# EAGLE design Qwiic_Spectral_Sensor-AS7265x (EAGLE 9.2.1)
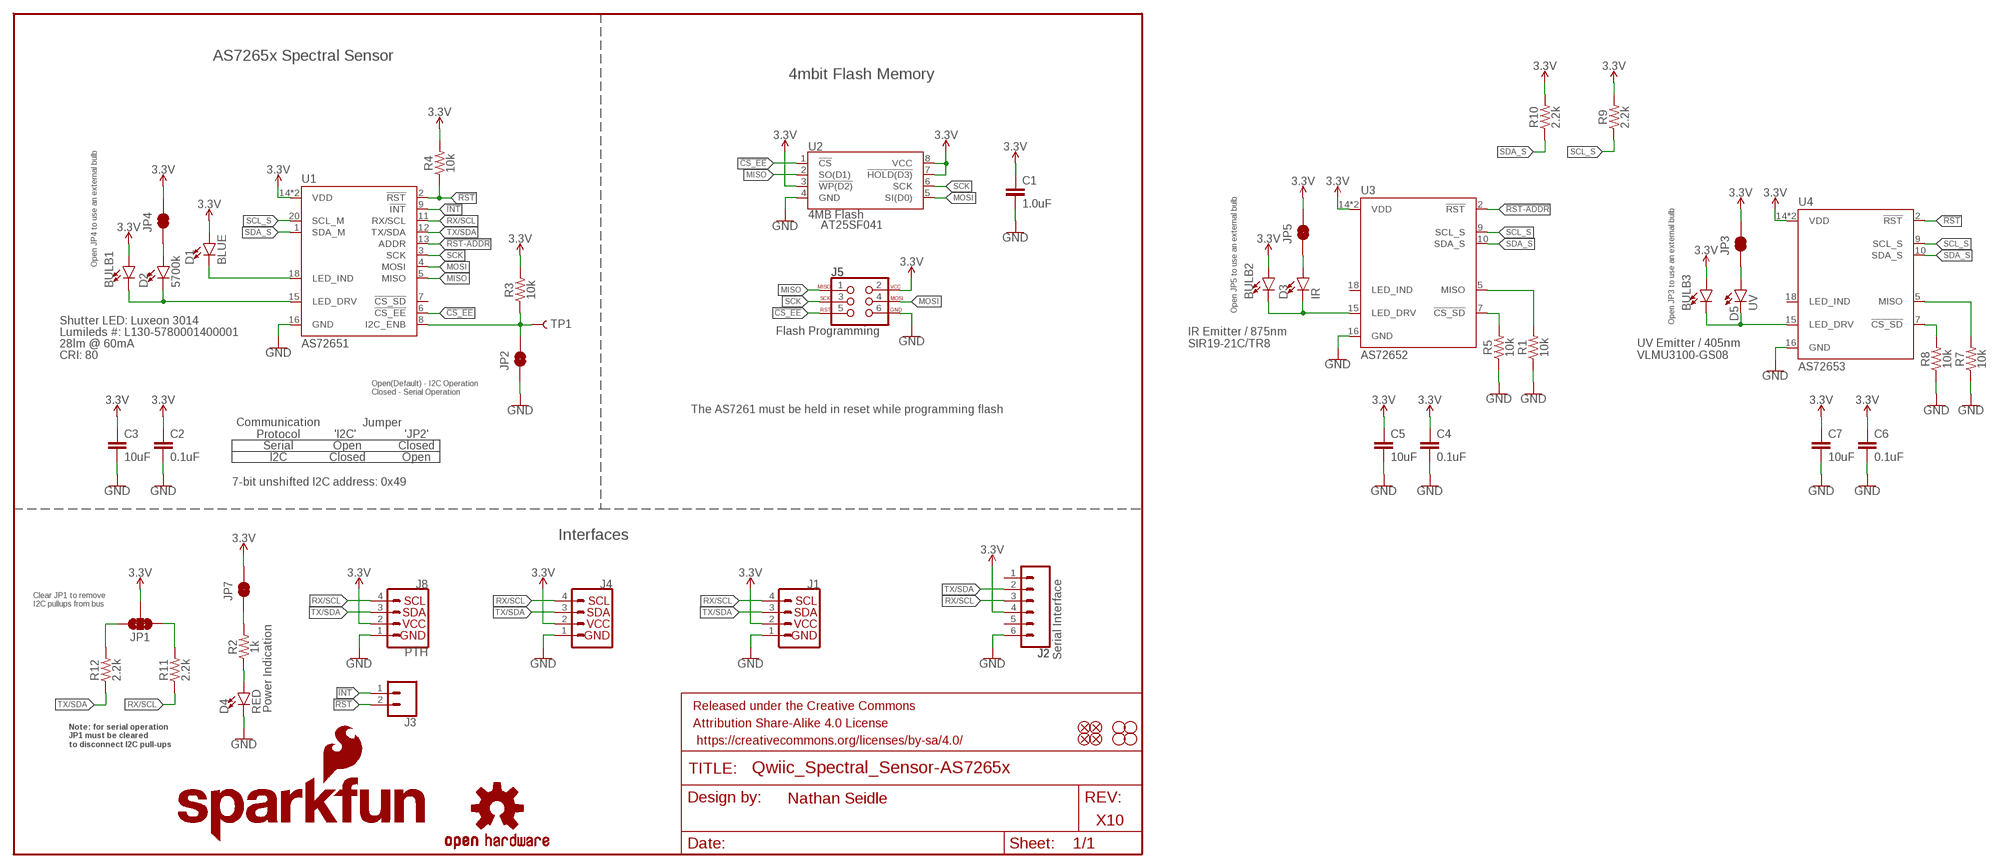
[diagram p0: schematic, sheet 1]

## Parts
BULB1  LEDNS  [LED_5MM_NOSILK]
BULB2  LEDNS  [LED_5MM_NOSILK]
BULB3  LEDNS  [LED_5MM_NOSILK]
C1  1.0uF  1.0UF-0603-16V-10%  [0603]
C2  0.1uF  0.1UF-0603-25V-(+80/-20%)  [0603]
C3  10uF  10UF-0603-6.3V-20%  [0603]
C4  0.1uF  0.1UF-0603-25V-(+80/-20%)  [0603]
C5  10uF  10UF-0603-6.3V-20%  [0603]
C6  0.1uF  0.1UF-0603-25V-(+80/-20%)  [0603]
C7  10uF  10UF-0603-6.3V-20%  [0603]
D1  BLUE  LED-BLUE0603  [LED-0603]
D2  5700k  LED-WHITE3014  [SUPER_BRIGHT_SMD_LED_3014]
D3  IR  LED-IR0603  [LED-0603]
D4  RED  LED-RED0603  [LED-0603]
D5  UV  LED-UVPLCC  [PLCC-2]
FD1  FIDUCIAL1X2  [FIDUCIAL-1X2]
FD2  FIDUCIAL1X2  [FIDUCIAL-1X2]
FD3  FIDUCIAL1X2  [FIDUCIAL-1X2]
FD4  FIDUCIAL1X2  [FIDUCIAL-1X2]
FRAME1  FRAME-LETTER  [CREATIVE_COMMONS]
H1  STAND-OFF  [STAND-OFF]
H2  STAND-OFF  [STAND-OFF]
H3  STAND-OFF  [STAND-OFF]
H4  STAND-OFF  [STAND-OFF]
J1  QWIIC_CONNECTORJS-1MM  [1X04_1MM_RA]
J2  Serial Interface  CONN_06NO_SILK_FEMALE_PTH  [1X06_NO_SILK]
J3  CONN_021X02_NO_SILK  [1X02_NO_SILK]
J4  QWIIC_CONNECTORJS-1MM  [1X04_1MM_RA]
J5  Flash Programming  AVR_SPI_PROG_3X2TESTPOINTS  [2X3_TEST_POINTS]
J8  PTH  I2C_STANDARD_NO_SILK  [1X04_NO_SILK]
JP1  JUMPER-SMT_3_2-NC_TRACE_SILK  [SMT-JUMPER_3_2-NC_TRACE_SILK]
JP2  JUMPER-SMT_2_NO_SILK  [SMT-JUMPER_2_NO_SILK]
JP3  JUMPER-SMT_2_NC_TRACE_NO-SILK  [SMT-JUMPER_2_NC_TRACE_NO-SILK]
JP4  JUMPER-SMT_2_NC_TRACE_NO-SILK  [SMT-JUMPER_2_NC_TRACE_NO-SILK]
JP5  JUMPER-SMT_2_NC_TRACE_NO-SILK  [SMT-JUMPER_2_NC_TRACE_NO-SILK]
JP7  JUMPER-SMT_2_NC_TRACE_NO-SILK  [SMT-JUMPER_2_NC_TRACE_NO-SILK]
LOGO1  SFE_LOGO_NAME_FLAME.1_INCH  [SFE_LOGO_NAME_FLAME_.1]
LOGO4  OSHW-LOGOS  [OSHW-LOGO-S]
R1  10k  10KOHM-0603-1/10W-1%  [0603]
R2  1k  1KOHM-0603-1/10W-1%  [0603]
R3  10k  10KOHM-0603-1/10W-1%  [0603]
R4  10k  10KOHM-0603-1/10W-1%  [0603]
R5  10k  10KOHM-0603-1/10W-1%  [0603]
R7  10k  10KOHM-0603-1/10W-1%  [0603]
R8  10k  10KOHM-0603-1/10W-1%  [0603]
R9  2.2k  2.2KOHM-0603-1/10W-1%  [0603]
R10  2.2k  2.2KOHM-0603-1/10W-1%  [0603]
R11  2.2k  2.2KOHM-0603-1/10W-1%  [0603]
R12  2.2k  2.2KOHM-0603-1/10W-1%  [0603]
TP1  TEST-POINT3  [PAD.03X.03]
U1  AS72651  [LGA20]
U2  4MB Flash  AT25SF041  [SO08]
U3  AS72652  [LGA20]
U4  AS72653  [LGA20]

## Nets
3.3V [Power]: BULB1.A BULB2.A BULB3.A C1.1 C2.1 C3.1 C4.1 C5.1 C6.1 C7.1 D1.A J1.2 J2.4 J4.2 J5.2 J8.2 JP1.2 JP3.2 JP4.2 JP5.2 JP7.2 R3.2 R4.2 R9.2 R10.2 U1.14(VDD) U1.17(VDD) U2.3(!WP(D2)) U2.7(!HOLD(D3)) U2.8(VCC) U3.14(VDD) U3.17(VDD) U4.14(VDD) U4.17(VDD)
!CS_EE: J5.5 U1.6(!CS_EE) U2.1(!CS)
!INT: J3.1 U1.9(!INT)
!RST: J3.2 R4.1 U1.2(!RST) U4.2(!RST)
!RST-ADDR: U1.13(ADDR) U3.2(!RST)
GND: C1.2 C2.2 C3.2 C4.2 C5.2 C6.2 C7.2 D4.C J1.1 J2.6 J4.1 J5.6 J8.1 JP2.1 R1.1 R5.1 R7.1 R8.1 U1.16(GND) U2.4(GND) U3.16(GND) U4.16(GND)
I2C_ENB: JP2.2 R3.1 TP1.P$1 U1.8(I2C_ENB)
LED_DRV: BULB1.K(C) D2.C U1.15(LED_DRV)
LED_DRV1: BULB2.K(C) D3.C U3.15(LED_DRV)
LED_DRV2: BULB3.K(C) D5.C U4.15(LED_DRV)
MISO: J5.1 U1.5(MISO) U2.2(SO(D1))
MOSI: J5.4 U1.4(MOSI) U2.5(SI(D0))
N$1: JP7.1 R2.2
N$2: D1.C U1.18(LED_IND)
N$3: R5.2 U3.7(!CS_SD)
N$4: JP1.3 R12.2
N$5: JP1.1 R11.2
N$6: D2.A JP4.1
N$7: D4.A R2.1
N$8: D3.A JP5.1
N$9: R1.2 U3.5(MISO)
N$11: D5.A JP3.1
N$12: R8.2 U4.7(!CS_SD)
N$13: R7.2 U4.5(MISO)
RX/SCL: J1.4 J2.3 J4.4 J8.4 R11.1 U1.11(RX/SCL)
SCK: J5.3 U1.3(SCK) U2.6(SCK)
SCL_S: R9.1 U1.20(SCL_M) U3.9(SCL_S) U4.9(SCL_S)
SDA_S: R10.1 U1.1(SDA_M) U3.10(SDA_S) U4.10(SDA_S)
TX/SDA: J1.3 J2.2 J4.3 J8.3 R12.1 U1.12(TX/SDA)
Unconnected: J2.1 J2.5 U1.7(!CS_SD) U3.18(LED_IND) U4.18(LED_IND)

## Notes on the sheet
- AS7265x Spectral Sensor
- 4mbit Flash Memory
- AT25SF041
- Open JP4 to use an external bulb
- Open JP5 to use an external bulb
- Shutter LED: Luxeon 3014 | Open JP3 to use an external bulb
- Lumileds #: L130-5780001400001
- 28lm @ 60mA
- IR Emitter / 875nm
  SIR19-21C/TR8
- CRI: 80
- UV Emitter / 405nm
  VLMU3100-GS08
- Open(Default) - I2C Operation
  Closed - Serial Operation
- The AS7261 must be held in reset while programming flash
- Jumper
- Communication
  Protocol
- 'I2C' | 'JP2'
- Serial | Open | Closed
- I2C | Closed | Open
- 7-bit unshifted I2C address: 0x49
- Interfaces
- Clear JP1 to remove
  I2C pullups from bus
- Power Indication
- Note: for serial operation
  JP1 must be cleared
  to disconnect I2C pull-ups
- Nathan Seidle
- X10

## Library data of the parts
BULB1-BULB3 = SparkX:LED
C1 = SparkFun-Capacitors:1.0UF: 1µF ceramic capacitors; PROD_ID: CAP-00868
C2 C4 C6 = SparkFun-Capacitors:0.1UF: 0.1µF ceramic capacitors; PROD_ID: CAP-00810
C3 C5 C7 = SparkFun-Capacitors:10UF: 10.0µF ceramic capacitors; PROD_ID: CAP-11015
D1 = SparkFun-LED:LED-BLUE: Blue SMD LED; PROD_ID: DIO-08575
D2 = SparkFun-LED:LED-WHITE: White SMD LED; PROD_ID: DIO-13728; VALUE: White, 60mA
D3 = SparkFun-LED:LED-IR: Infrared LED (IR); PROD_ID: DIO-14125
D4 = SparkFun-LED:LED-RED: Red SMD LED; PROD_ID: DIO-00819
D5 = SparkFun-LED:LED-UV; PROD_ID: DIO-14126
FD1-FD4 = SparkFun-Aesthetics:FIDUCIAL: Fiducial Alignment Points
FRAME1 = SparkFun-Aesthetics:FRAME-LETTER: Schematic Frame - Letter
H1-H4 = SparkFun-Hardware:STAND-OFF: Stand Off
J1 J4 = SparkFun-Connectors:QWIIC_CONNECTOR: SparkFun I2C Standard Qwiic Connector An SMD 1mm pitch JST connector makes it easy and quick (get it? Qwiic?) to connect I2C devices to each other. The Qwiic system enables fast and solderless connection between popular platforms and various sensors and actuators. We carry 200mm, 100mm, 50mm, and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; PROD_ID: CONN-13694
J2 = SparkFun-Connectors:CONN_06: Multi connection point. Often used as Generic Header-pin footprint for 0.1 inch spaced/style header connections On any of the 0.1 inch spaced packages, you can populate with these: Break Away Headers - Straight (PRT-00116) Break Away Male Headers - Right Angle (PRT-00553) Female Headers (PRT-00115)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; PROD_ID: CONN-08437
J3 = SparkFun-Connectors:CONN_02: Multi connection point. Often used as Generic Header-pin footprint for 0.1 inch spaced/style header connections
J5 = SparkFun-Connectors:AVR_SPI_PROG_3X2: AVR ISP 6 Pin This is the reduced ISP connector for AVR programming. Common on Arduino. This footprint will take up less PCB space and can be used with a 10-pin to 6-pin adapter such as SKU: BOB-08508 **Special note about "TEST_POINT" package. The stop mask is on the top side, so if you want your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
J8 = SparkFun-Connectors:I2C_STANDARD: SparkFun I2C Standard Pinout Header SparkFun has standardized on a pinout for all I2C based sensor breakouts. This pinout allows I2C boards to be plugged directly into the headers on Arduino Uno compatible boards, and to be daisy chained easily. Example SparkFun Products: SparkFun Atmospheric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
JP1 = SparkFun-Jumpers:JUMPER-SMT_3_2-NC_TRACE: Normally closed trace jumper (2 of 2 connections) This jumper has a trace between all three pads so they are normally closed (NC). Use a razor knife to open the connection(s). For best results follow the IPC guidelines for cutting traces: Cutout at least 0.063 mm (0.005 in). Remove all loose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
JP2 = SparkFun-Jumpers:JUMPER-SMT_2_NO: Normally open jumper
JP3-JP5 JP7 = SparkFun-Jumpers:JUMPER-SMT_2_NC_TRACE: Normally closed trace jumper
LOGO1 = SparkFun-Aesthetics:SFE_LOGO_NAME_FLAME: SparkFun Font Logo w/ Flame
LOGO4 = SparkFun-Aesthetics:OSHW-LOGO: Open-Source Hardware (OSHW) Logo
R1 R3-R5 R7 R8 = SparkFun-Resistors:10KOHM: 10kΩ resistor; PROD_ID: RES-00824
R2 = SparkFun-Resistors:1KOHM: 1kΩ resistor; PROD_ID: RES-07856
R9-R12 = SparkFun-Resistors:2.2KOHM: 2.2kΩ resistor; PROD_ID: RES-08272
TP1 = SparkFun-Connectors:TEST-POINT: SparkFun Test Points
U1 = Qwiic_Spectral_Sensor-AS7265x:AS72651; PROD_ID: IC-14127
U2 = SparkFun-IC-Memory:AT25SF041: AT25SF041 4Mb Serial Flash Memory 104MHz, SPI, 8-SOIC Datasheet SparkFun Products: SparkFun ESP8266 Thing SparkFun ESP8266 Thing - Dev Board; PROD_ID: IC-12455
U3 = Qwiic_Spectral_Sensor-AS7265x:AS72652; PROD_ID: IC-14128
U4 = Qwiic_Spectral_Sensor-AS7265x:AS72653; PROD_ID: IC-14129

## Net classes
1 Power: width 0.305 mm

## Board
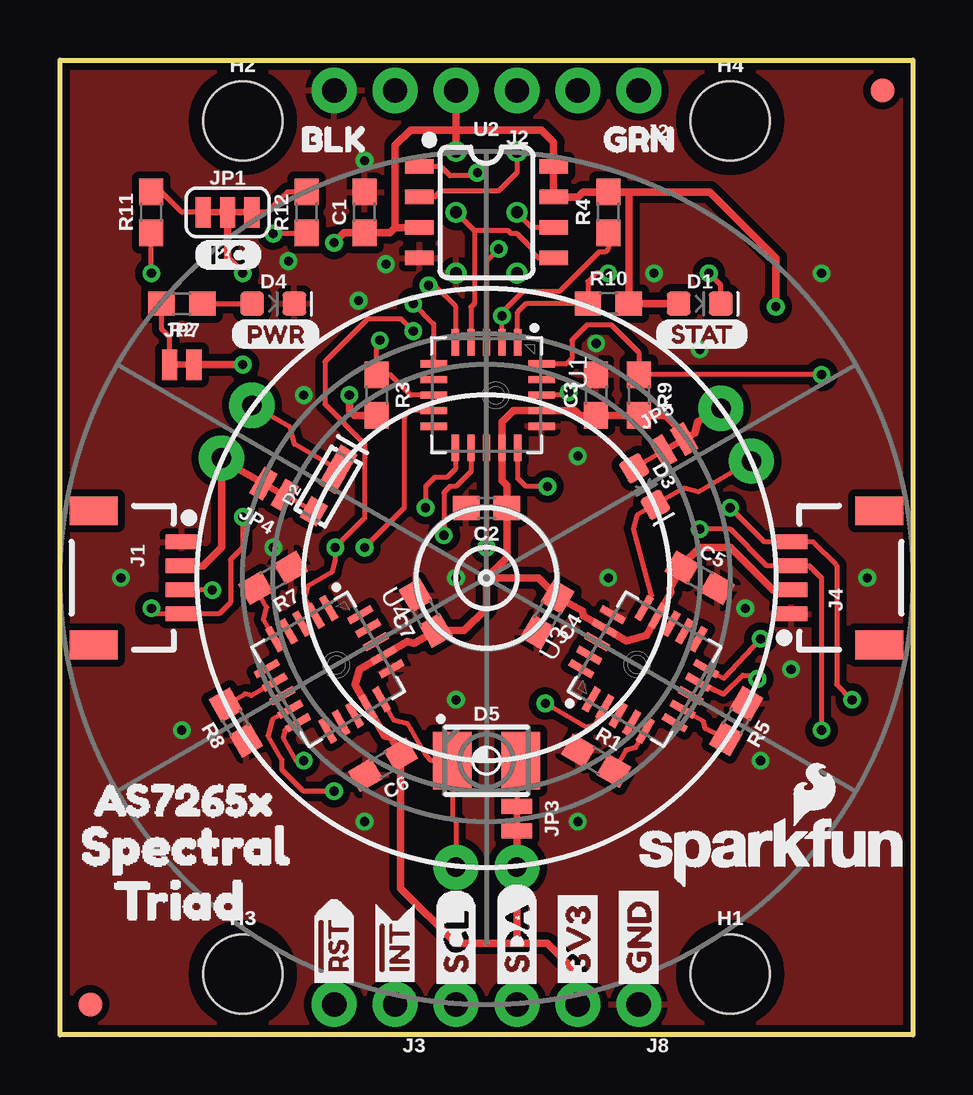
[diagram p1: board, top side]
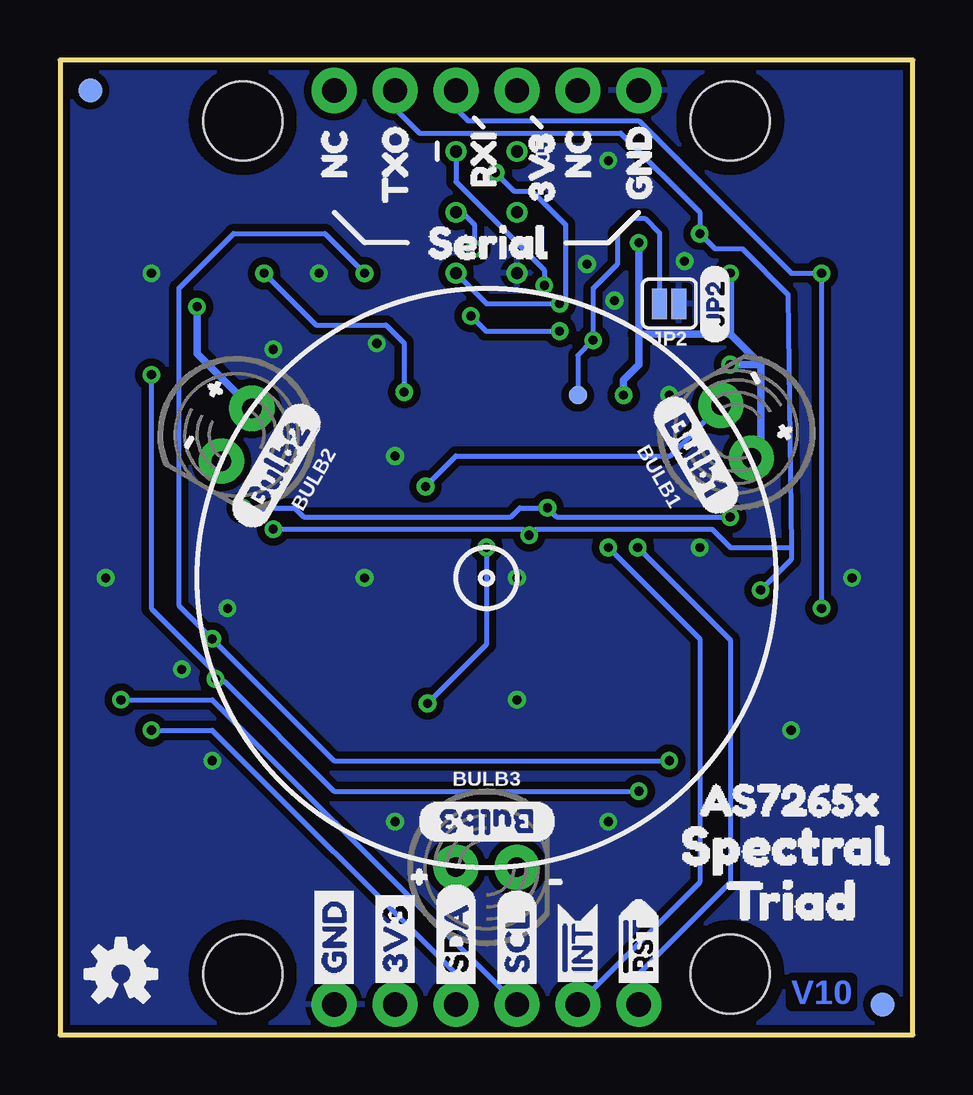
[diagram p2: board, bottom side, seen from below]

Size 35.56 x 40.64 mm. Coordinates in mm from the lower left corner, seen from the top.
Outline: 0,0 0,40.64 35.56,40.64 35.56,0 0,0
Copper layers (1*16): Top 0.035mm / dielectric 1.5mm / Bottom 0.035mm
Design rules "SparkFun-2-layer-TIGHT *": minimum track width 7mil, minimum drill 15mil, track to track 7mil, track to pad 7mil, pad to pad 7mil, via to via 7mil, smd to smd 7mil, copper to edge 7mil, drill to drill 7mil, minimum pad ring 7mil, minimum via ring 7mil, stop-mask expansion 4mil, vias tented up to drill 25mil, thermal gap 10mil

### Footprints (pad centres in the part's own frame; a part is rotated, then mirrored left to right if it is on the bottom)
LED_5MM_NOSILK = drill 0.813 pad 1.88: A -1.27,0; K 1.27,0
0603 = smd 1.1 x 1: 1 -0.85,0; 2 0.85,0
LED-0603 = smd 1 x 1: A -0.877,0; C 0.877,0
SUPER_BRIGHT_SMD_LED_3014 = smd 1 x 0.8: A -1.2,0 | smd 1.9 x 0.8: C 0.827,0
PLCC-2 = smd 1.6 x 2.4: A 1.425,0; C -1.425,0
FIDUCIAL-1X2 = smd 1 x 1: 1 0,0
STAND-OFF = hole 3.302: 0,0
1X04_1MM_RA = smd 0.6 x 1.35: 1 -1.5,0; 2 -0.5,0; 3 0.5,0; 4 1.5,0 | smd 1.2 x 2: NC1 2.8,-3.675; NC2 -2.8,-3.675
1X06_NO_SILK = drill 1.016 pad 1.88: 1 0,0; 2 2.54,0; 3 5.08,0; 4 7.62,0; 5 10.16,0; 6 12.7,0
1X02_NO_SILK = drill 1.016 pad 1.88: 1 0,0; 2 2.54,0
2X3_TEST_POINTS = drill 0.508: 1 -2.54,-1.27; 2 -2.54,1.27; 3 0,-1.27; 4 0,1.27; 5 2.54,-1.27; 6 2.54,1.27
1X04_NO_SILK = drill 1.016 pad 1.88: 1 0,0; 2 2.54,0; 3 5.08,0; 4 7.62,0
SMT-JUMPER_3_2-NC_TRACE_SILK = smd 0.635 x 1.27: 1 -1.016,0; 2 0,0; 3 1.016,0
SMT-JUMPER_2_NO_SILK = smd 0.635 x 1.27: 1 -0.406,0; 2 0.406,0
SMT-JUMPER_2_NC_TRACE_NO-SILK = smd 0.635 x 1.27: 1 -0.508,0; 2 0.508,0
PAD.03X.03 = smd 0.762 x 0.762: P$1 0,0
LGA20 = smd 1.1 x 0.3: 1 -2.2,1.3; 2 -2.2,0.65; 3 -2.2,0; 4 -2.2,-0.65; 5 -2.2,-1.3; 11 2.2,-1.3; 12 2.2,-0.65; 13 2.2,0; 14 2.2,0.65; 15 2.2,1.3 | smd 0.3 x 1.1: 6 -1.3,-2.2; 7 -0.65,-2.2; 8 0,-2.2; 9 0.65,-2.2; 10 1.3,-2.2; 16 1.3,2.3; 17 0.65,2.3; 18 0,2.3; 19 -0.65,2.3; 20 -1.3,2.3
SO08 = smd 0.6 x 1.2: 1 -1.905,-2.8; 2 -0.635,-2.8; 3 0.635,-2.8; 4 1.905,-2.8; 5 1.905,2.8; 6 0.635,2.8; 7 -0.635,2.8; 8 -1.905,2.8

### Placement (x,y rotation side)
BULB1  7.37,25.15 120 bottom
BULB2  28.19,25.02 240 bottom
BULB3  17.78,6.99 0 bottom
C1  12.7,34.29 90 top
C2  17.78,21.97 180 top
C3  22.35,26.67 90 top
C4  20.32,17.53 240 top
C5  26.67,19.05 330 top
C6  13.47,11.26 210 top
C7  15.25,17.59 120 top
D1  26.67,30.48 0 top
D2  11.18,22.86 60 top
D3  24.38,22.86 300 top
D4  8.89,30.48 0 top
D5  17.78,11.43 0 top
FD1  1.27,1.27 0 top
FD2  34.29,39.37 0 top
FD3  34.29,39.37 0 bottom
FD4  1.27,1.27 0 bottom
FRAME1  not placed on the board
H1  27.94,2.54 0 top
H2  7.62,38.1 0 top
H3  7.62,2.54 0 top
H4  27.94,38.1 0 top
J1  5.08,19.05 270 top
J2  24.13,39.37 180 top
J3  13.97,1.27 180 top
J4  30.48,19.05 90 top
J5  17.78,34.29 270 bottom
J8  24.13,1.27 180 top
JP1  6.98,34.29 0 top
JP2  10.16,30.48 180 bottom
JP3  19.05,9.02 270 top
JP4  8.93,22.73 150 top
JP5  25.58,24.58 30 top
JP7  5.08,27.94 0 top
LOGO1  29.72,7.62 0 top
LOGO4  33.02,2.54 0 bottom
R1  22.35,11.43 330 top
R2  5.08,30.48 180 top
R3  13.21,26.67 270 top
R4  22.86,34.29 90 top
R5  28.19,13.08 240 top
R7  8.89,19.05 210 top
R8  7.33,13.02 120 top
R9  24.13,26.67 270 top
R10  22.86,30.48 0 top
R11  3.81,34.29 90 top
R12  10.29,34.29 90 top
TP1  13.97,26.67 0 bottom
U1  17.78,26.67 270 top
U2  17.78,34.29 270 top
U3  24.38,15.24 60 top
U4  11.18,15.24 300 top
U$1  [#0]  29.84,25.91 60 bottom
U$2  [I_SUPER2_C-()-03]  5.59,32.51 0 top
U$3  [PWR-()-03]  7.11,29.21 0 top
U$4  [AS7265X0]  0.25,9.78 0 top
U$5  [BULB15]  10.41,26.54 300 bottom
U$6  [BULB26]  28.07,21.08 60 bottom
U$7  [BULB37]  14.86,8.89 180 bottom
U$8  [JP20]  8.25,28.83 90 bottom
U$9  [SPECTRAL1]  -0.51,7.87 0 top
U$10  [STAT4]  24.76,29.21 0 top
U$11  [TRIAD2]  0.89,5.59 0 top
U$12  [TRIAD2]  9.14,5.59 0 bottom
U$13  [SPECTRAL1]  11.05,7.87 0 bottom
U$14  [AS7265X0]  10.03,9.78 0 bottom
U$15  [3V33]  15.49,33.65 90 bottom
U$16  [BLK7]  9.14,37.34 0 top
U$17  [GND5]  11.43,33.91 90 bottom
U$18  [GRN6]  21.59,37.34 0 top
U$19  [NC4]  24.13,34.8 90 bottom
U$20  [NC4]  13.97,34.8 90 bottom
U$21  [RXI2]  17.91,34.42 90 bottom
U$22  [SERIAL0]  21.34,33.02 0 bottom
U$23  [TXO1]  21.59,33.78 90 bottom
U$24  [3V3-04]  21.59,1.65 90 bottom
U$25  [GND-04]  24.13,1.65 90 bottom
U$26  [SDA-[)]  19.05,1.65 90 bottom
U$27  [SCL-[)]  16.51,1.65 90 bottom
U$28  [INT#-[<-04]  13.97,1.52 90 bottom
U$29  [RST#-[>-04]  11.43,1.52 90 bottom
U$30  [GND-04]  24.13,1.65 90 top
U$31  [3V3-04]  21.59,1.65 90 top
U$32  [SDA-[)]  19.05,1.65 90 top
U$33  [SCL-[)]  16.51,1.65 90 top
U$34  [INT#-[<-04]  13.97,1.52 90 top
U$35  [RST#-[>-04]  11.43,1.52 90 top
U$36  [#0]  5.84,26.29 300 bottom
U$37  [#0]  21.84,6.73 0 bottom
U$38  [#1]  16.13,6.6 0 bottom
U$39  [#1]  6.98,28.57 300 bottom
U$40  [#1]  30.99,23.75 60 bottom

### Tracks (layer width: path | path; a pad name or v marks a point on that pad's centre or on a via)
3.3V  (via drill 0.38)
  Top 0.203: 25.78,30.49 D1.A
  Top 0.305: U2.3 13.97,33.65 | 20.32,37.46 20.58,37.2 U2.8 U2.7 21.59,34.92 21.8,35.14 R4.2 23.75,35.14 | BULB2.A 26.59,25.56 26.46,25.09 JP5.2 26.02,25.03 25.23,25.82 R9.2 C3.1 21.68,25.82 21.48,26.02 U1.17 18.91,26.02 18.43,25.54 U1.14 18.43,23.1 18.63,22.9 C2.1 18.63,19.9 17.78,19.05 | JP3.2 BULB3.A 19.05,3.81 | JP4.2 6.75,23.99 6.73,24 BULB1.A 6.73,20.32 5.96,19.55 J1.2 | J4.2 29.71,18.55 27.94,20.32 26.67,20.32 25.93,19.58 C5.1 25.43,18.6 25.47,18.44 U3.14 24.44,16.65 23.62,16.43 U3.17 21.83,17.46 21.78,17.67 C4.1 19.96,19.05 17.78,19.05 | 25.78,35.14 23.75,35.14 | 25.78,35.14 27.09,35.14 29.84,32.38 v29.84,30.35 | v11.43,33.02 11.85,33.44 C1.1 13.75,33.44 13.97,33.65 | R3.2 12.28,25.82 12.06,26.03 v12.06,26.67 | 17.78,19.05 17.78,17.78 16.85,16.85 C7.1 14.76,16.33 14.49,16.4 U4.17 12.48,15.24 12.31,14.59 U4.14 13.53,12.47 13.79,12.4 C6.1 14.21,6.11 16.51,3.81 19.05,3.81 | 20.32,37.46 20.07,37.72 | 16,37.72 14.6,37.72 13.97,37.08 13.97,33.65 | 19.05,3.81 20.32,3.81 21.59,2.54 J8.2 | v7.62,31.75 6.98,32.38 JP1.2 | 25.79,35.13 25.78,35.14 | 20.32,37.46 | 16,37.72 | 16.51,37.72 16,37.72 | 20.07,37.72 16.51,37.72 | 20.07,37.72 | J2.4 16.51,37.72 | 16.51,37.72 | 16.51,37.72 J5.2 | J8.2 | JP7.2 v7.62,27.94 | R10.2 23.71,35.1 23.75,35.14 | D1.A R10.2 | R10.2
  Bottom 0.305: v29.84,30.35 29.84,28.4 BULB2.A | 11.43,29.21 7.62,29.21 | 7.62,29.21 6.35,27.94 | 6.35,27.94 6.35,24.43 BULB1.A | v11.43,33.02 11.43,29.21 | 11.43,29.21 11.43,27.94 12.06,27.3 v12.06,26.67 | v7.62,31.75 7.62,29.21 | v7.62,27.94 6.35,27.94
!CS_EE  (via drill 0.38)
  Top 0.203: U1.6 15.58,29.63 v14.73,30.48 | U2.1 15.87,36.19 16.26,35.81 17.27,35.81 v17.4,35.94
  Bottom 0.203: J5.5 17.78,30.48 v14.73,30.48 14.48,30.73 14.48,33.78 15.87,35.18 16.64,35.18 v17.4,35.94
!INT  (via drill 0.38)
  Top 0.203: U1.9 14.59,26.02 14.35,25.78 14.35,21.97 v12.7,20.32
  Bottom 0.203: J3.1 | J3.1 8.89,6.35 8.89,16.51 v12.7,20.32
!RST  (via drill 0.38)
  Top 0.203: U1.2 v18.43,29.97 18.43,30.11 19.3,30.99 20.83,30.99 22.48,32.64 22.73,32.64 22.86,32.77 R4.1 | v14.73,29.34 14.22,29.84 12.83,29.84 11.05,28.07 11.05,26.29 12.7,24.64 12.7,21.54 v11.48,20.32 11.48,19.81 11.34,19.29 10.35,18.72 10.21,18.22 U4.2
  Bottom 0.203: v18.43,29.97 17.79,29.34 v14.73,29.34 | v11.48,20.32 7.62,16.46 7.62,6.35 11.43,2.54 J3.2
!RST-ADDR  (via drill 0.38)
  Top 0.203: v20.23,13.82 21.96,12.82 22.28,12.91 U3.2 | U1.13 v17.78,20.32
  Bottom 0.203: v17.78,20.32 17.78,16.27 v20.23,13.82
GND  (via drill 0.38)
  other vias: 2.54,19.05 8.89,20.32 16.51,19.05 16.51,13.97 22.86,19.05 21.59,24.13 22.35,28.83 12.7,36.45 13.59,32.13 31.75,31.75 30.48,15.24 9.52,32.26 12.7,8.89 5.08,12.7 10.16,26.67 26.67,28.57 28.57,17.78 33.65,19.05 24.76,31.75 12.45,30.61 21.59,8.89 29.21,11.43
  pour Top (isolate 0.305): 0,0 35.56,0 35.56,40.64 0,40.64
  pour Bottom (isolate 0.305): 35.56,40.64 0,40.64 0,0 35.56,0
I2C_ENB  (via drill 0.38)
  Top 0.203: U1.8 14.6,26.67 13.75,27.52 R3.1 13.21,28.83 v13.33,28.96
  Bottom 0.203: JP2.2 10.57,33.43 11.18,34.04 11.68,34.04 12.32,33.4 12.32,32.13 13.33,31.11 v13.33,28.96 13.97,28.32 TP1.P$1
LED_DRV  (via drill 0.38)
  Top 0.203: BULB1.K 9.59,25.33 9.78,24.62 D2.C | U1.15 19.08,23.21 19.43,22.86 v20.32,22.86
  Bottom 0.203: v20.32,22.86 19.05,24.13 10.12,24.13 BULB1.K
LED_DRV1
  Top 0.203: BULB2.K 26.6,22.63 26.02,22.79 D3.C 24.06,21.66 23.91,21.12 24.66,18.33 U3.15
LED_DRV2
  Top 0.203: BULB3.K 16.51,8.89 16.35,9.04 D5.C | U4.15 13.91,13.11 14.51,12.95 15.24,11.68 15.49,11.43 D5.C | D5.C
MISO  (via drill 0.38)
  Top 0.203: U1.5 16.48,29.11 16.48,30.38 15.62,31.24 v15.37,31.24 | J5.1 19.05,35.94 18.54,35.43 18.29,35.18 15.87,35.18 15.62,34.92 U2.2 | J5.1
  Bottom 0.203: v15.37,31.24 15.37,31.88 19.05,35.56 J5.1
MOSI
  Top 0.203: J5.4 17.13,33.67 17.27,33.53 | U1.4 17.13,30.34 17.27,30.48 17.27,33.53 | U2.5 19.94,32.38 19.68,32.64 19.68,32.77 19.05,33.4 18.8,33.4 18.67,33.53 17.27,33.53 | 17.27,33.53
N$1
  Top 0.203: JP7.1 4.57,29.08 4.23,29.42 R2.2
N$2  (via drill 0.38)
  Top 0.203: D1.C 27.55,31.25 v27.05,31.75 | U1.18 21.21,26.67 v21.21,26.8
  Bottom 0.203: v21.21,26.8 21.21,28.83 21.97,29.59 24.89,29.59 v27.05,31.75
N$3
  Top 0.203: U3.7 26.82,13.08 26.9,12.77 R5.2
N$4
  Top 0.203: JP1.3 8.64,34.29 9.49,35.14 R12.2
N$5
  Top 0.203: R11.2 4.23,35.14 5.08,34.29 JP1.1
N$6
  Top 0.203: JP4.1 9.42,22.49 D2.A
N$7
  Top 0.203: R2.1 D4.A
N$8
  Top 0.203: JP5.1 D3.A
N$9
  Top 0.203: R1.2 23.58,11.87 24,11.98 U3.5
N$11
  Top 0.203: 19.05,11.43 JP3.1 | 19.05,11.43 | D5.A 19.05,11.43
N$12
  Top 0.203: U4.7 7.98,14.14 7.71,14.22 R8.2
N$13
  Top 0.203: R7.2 8.62,17.82 8.48,17.31 U4.5
RX/SCL  (via drill 0.38)
  Top 0.203: v3.81,31.75 R11.1 | U1.11 16.48,23.59 16.13,23.24 15.62,23.24 15.24,22.86 v15.24,21.97 | v27.94,21.97 29.36,20.55 J4.4 31.39,20.55 32.38,19.56 32.38,14.6 v33.02,13.97 | v7.62,21.59 7.62,20.32 7.11,19.81 7.11,18.03 6.63,17.55 J1.4 4.04,17.55 v3.81,17.78
  Bottom 0.203: J2.3 19.05,38.61 18.54,38.1 11.43,38.1 5.08,31.75 v3.81,31.75 | v3.81,31.75 v3.81,17.78 | v3.81,17.78 | v27.94,21.97 25.78,21.97 25.4,21.59 16.76,21.59 16.38,21.97 v15.24,21.97 14.86,21.59 v7.62,21.59 | v3.81,31.75 | v33.02,13.97 29.21,13.97 19.05,3.81 | 19.05,3.81 | 19.05,3.81 J8.4
SCK  (via drill 0.38)
  Top 0.203: U2.6 19.68,33.65 J5.3 | U1.3 17.78,32.26 v18.29,32.77
  Bottom 0.203: J5.3 18.8,34.29 18.29,33.78 v18.29,32.77
SCL_S  (via drill 0.38)
  Top 0.203: 23.37,29.21 24.13,28.45 R9.1 | U1.20 21.11,27.97 21.34,28.19 21.34,28.96 21.59,29.21 21.97,29.59 22.99,29.59 23.37,29.21 | v31.75,27.52 R9.1 | R9.1 | v11.43,10.16 10.16,10.16 9.24,11.08 9.24,11.48 8.67,12.47 8.85,13.14 U4.9 | v29.08,14.84 28.93,14.99 28.45,14.99 27.67,14.2 U3.9 | 23.37,29.21
  Bottom 0.203: v11.43,10.16 24.13,10.16 28.69,14.72 28.96,14.72 v29.08,14.84 29.06,14.85 29.06,15.09 31.75,17.78 v31.75,27.52
SDA_S  (via drill 0.38)
  Top 0.203: U1.1 19.08,30.13 19.43,30.48 R10.1 22.01,31.41 22.35,31.75 v22.86,31.75 | v10.16,11.43 10.14,11.41 9.87,11.41 9.3,12.4 9.38,12.7 U4.10 | v29.21,16.51 27.69,14.86 U3.10
  Bottom 0.203: v22.86,31.75 24.51,33.4 28.32,33.4 30.61,31.11 30.61,17.91 v29.21,16.51 24.13,11.43 v10.16,11.43
TX/SDA  (via drill 0.38)
  Top 0.203: U1.12 17.13,23.48 16.51,22.86 16.26,22.86 16,22.61 v16,20.83 | v26.67,21.08 27.94,21.08 29.47,19.55 J4.3 31.25,19.55 31.75,19.05 v31.75,12.7 | J1.3 5.85,18.55 v6.35,18.54 | R12.1 10.25,33.4 v8.89,33.4
  Bottom 0.203: J2.2 21.59,38.61 20.57,37.59 12.19,37.59 8.89,34.29 v8.89,33.4 8.25,32.77 7.11,32.77 5.21,30.86 5.08,20.32 | 5.08,20.32 5.08,19.81 v6.35,18.54 | J8.3 19.05,2.54 29.21,12.7 v31.75,12.7 | 5.08,20.32 7.62,20.32 8.38,21.08 15.75,21.08 v16,20.83 16.26,21.08 v26.67,21.08

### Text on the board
Bottom: V10
tDocu: Nathan Seidle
